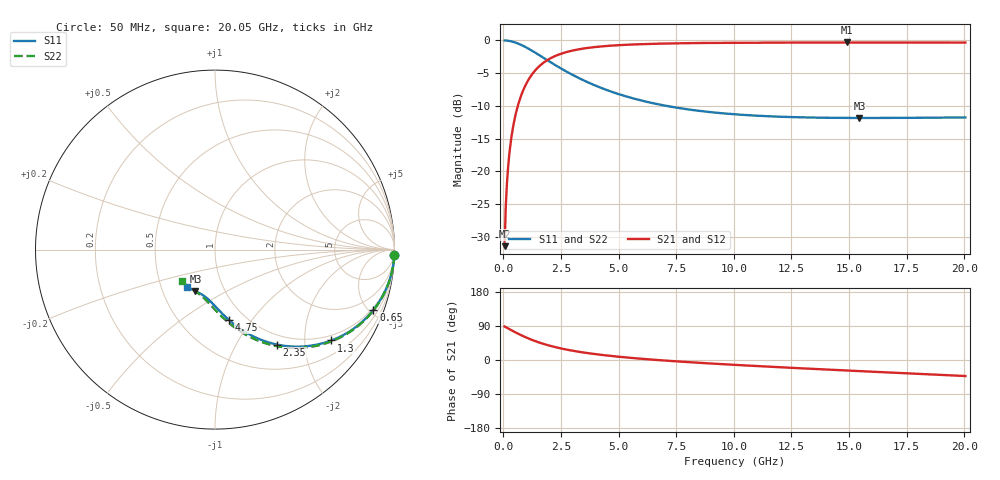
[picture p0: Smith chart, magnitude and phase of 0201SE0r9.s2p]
! AVX Thin Film Operation		Date: August 2001
! Description: Accu-P® Series, Thin Film, SMD, RF Capacitor
! Part Number: 02013J0R9ABW
! 50 MHz  -  20.05 GHz
! Serial Measurements
# mhz S db R 50
!	S11		S21		S12		S22
!	dB	Phase	dB	Phase	dB	Phase	dB	Phase
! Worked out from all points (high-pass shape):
!   401 points, 50 MHz to 20.05 GHz, reference 50 ohm
!   highest |S21| = -0.31 dB at 14.9 GHz (marker M1); lowest = -31.4 dB at 50 MHz (marker M2)
!   |S21| within 3 dB of the highest: 1.774 GHz to end of sweep
!   lowest |S11| = -11.8 dB at 15.45 GHz (marker M3), VSWR 1.69, Z = 36.4 - j18 ohm
!   |S11| at or under -10 dB: 7.07 GHz to end of sweep
!   |S22| runs from -11.9 to 0.0 dB; largest |S21 - S12| = 0
!   S11 on the Smith chart (normalised r, x): 50 MHz: 1, -69; 650 MHz: 0.85, -5.30; 1.3 GHz: 0.85, -2.66; 2.35 GHz: 0.85, -1.50; 4.75 GHz: 0.84, -0.79; 20.05 GHz: 0.68, -0.30
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50  -0.00 -1.7  -31.44 88.3  -31.44 88.3  -0.00 -1.7
100  -0.01 -3.3  -25.43 86.7  -25.43 86.7  -0.01 -3.4
200  -0.05 -6.6  -19.45 83.3  -19.45 83.3  -0.05 -6.7
250  -0.08 -8.3  -17.54 81.6  -17.54 81.6  -0.08 -8.4
300  -0.11 -9.9  -15.99 80.0  -15.99 80.0  -0.11 -10.1
450  -0.25 -14.7  -12.61 75.2  -12.61 75.2  -0.25 -14.9
650  -0.50 -20.9  -9.67 69.0  -9.67 69.0  -0.50 -21.2
950  -0.99 -29.3  -6.90 60.4  -6.90 60.4  -0.99 -29.8
1300  -1.70 -38.0  -4.91 51.6  -4.91 51.6  -1.70 -38.7
1750  -2.68 -47.2  -3.38 42.3  -3.38 42.3  -2.68 -48.1
2350  -3.98 -56.8  -2.23 32.5  -2.23 32.5  -3.98 -58.0
2850  -4.98 -63.0  -1.67 26.2  -1.67 26.2  -4.98 -64.5
3400  -5.97 -68.5  -1.28 20.5  -1.28 20.5  -5.97 -70.3
4050  -6.99 -73.8  -0.98 15.0  -0.98 15.0  -6.99 -75.9
4750  -7.91 -78.5  -0.78 10.2  -0.78 10.2  -7.91 -80.9
6750  -9.78 -88.4  -0.49 -0.3  -0.49 -0.3  -9.79 -91.8
10050  -11.29 -100.0  -0.35 -12.9  -0.35 -12.9  -11.31 -104.9
13400  -11.79 -109.7  -0.32 -23.3  -0.32 -23.3  -11.82 -116.0
14900  -11.84 -113.8  -0.32 -27.7  -0.32 -27.7  -11.88 -120.7
15450  -11.85 -115.2  -0.32 -29.3  -0.32 -29.3  -11.89 -122.4
16750  -11.84 -118.6  -0.32 -33.0  -0.32 -33.0  -11.89 -126.4
20050  -11.77 -127.1  -0.33 -42.3  -0.33 -42.3  -11.83 -136.3
